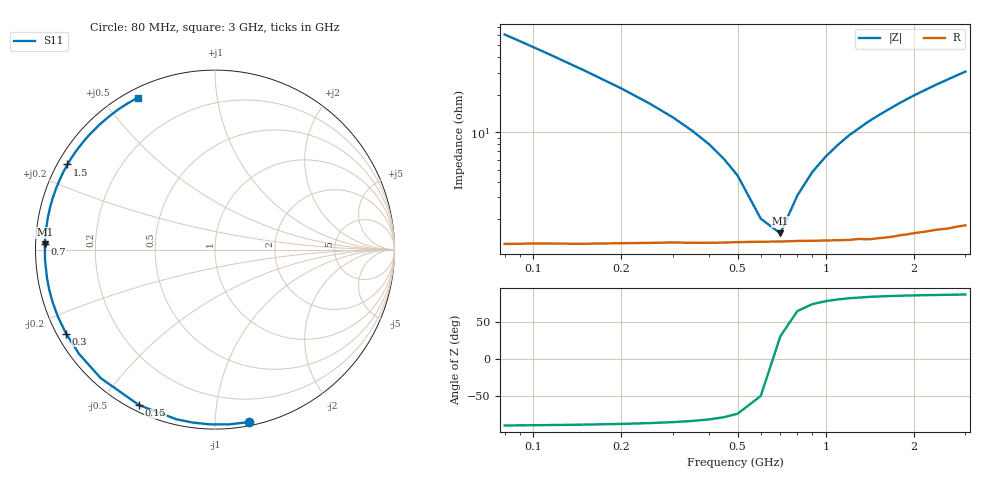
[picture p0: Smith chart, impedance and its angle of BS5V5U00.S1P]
! SIEMENS Small Signal Semiconductors
! BB640
! Si Tuning Diode in SOD323
! VR = 5.5 V
! S-Parameters:  July  1993
# GHz  S  MA  R  50
!  f  S11
! GHz  MAG  ANG
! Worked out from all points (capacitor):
!   33 points, 80 MHz to 3 GHz, reference 50 ohm
!   read as one part to ground: C = 32.2 pF near 80 MHz
!   lowest |Z| = 1.54 ohm at 700 MHz (marker M1)
!   series resonance near 666 MHz, so ESL is about 1.8 nH
!   S11 on the Smith chart (normalised r, x): 80 MHz: 0.03, -1.22; 150 MHz: 0.03, -0.62; 300 MHz: 0.03, -0.26; 700 MHz: 0.03, +0.02; 1.5 GHz: 0.03, +0.27; 3 GHz: 0.04, +0.61
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0.08  0.9799 -78.7
0.09  0.9769 -85.6
0.1  0.974 -91.9
0.11  0.9716 -97.6
0.12  0.9694 -102.9
0.15  0.9642 -116.0
0.2  0.9583 -131.6
0.25  0.9549 -142.5
0.3  0.9526 -150.6
0.35  0.9517 -157.0
0.4  0.9509 -162.1
0.45  0.9502 -166.5
0.5  0.9495 -170.2
0.6  0.9488 -176.5
0.7  0.9486 178.2
0.8  0.9482 173.6
0.9  0.9483 169.5
1  0.9484 165.8
1.2  0.9488 158.9
1.4  0.9494 152.8
1.5  0.9491 150.0
1.6  0.949 147.3
1.8  0.9483 142.0
2  0.948 137.1
2.2  0.9481 132.6
2.4  0.9481 128.3
2.8  0.9489 120.6
3  0.9495 117.0
